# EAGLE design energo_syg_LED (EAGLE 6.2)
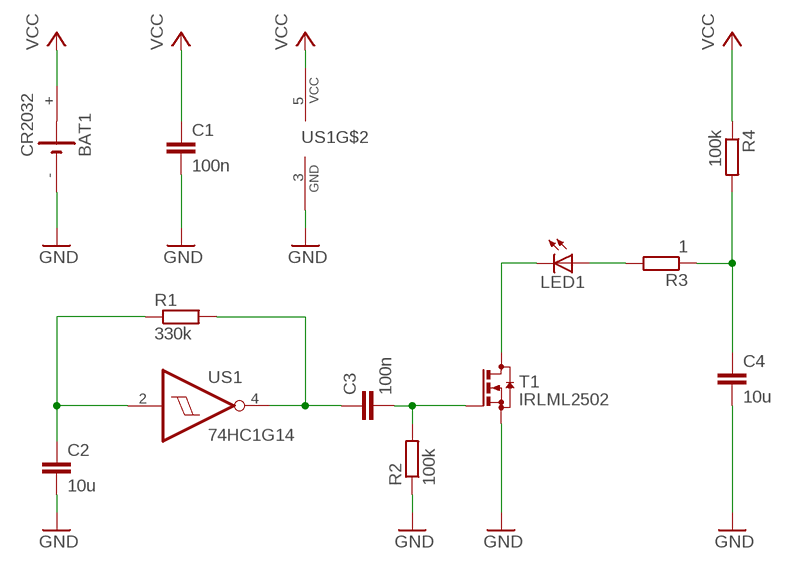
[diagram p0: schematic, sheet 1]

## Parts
BAT1  CR2032  BAT_20/16_XX  [BAT_CR2032]
C1  100n  C-EUC0805  [C0805]
C2  10u  C-EUC0805  [C0805]
C3  100n  C-EUC0805  [C0805]
C4  10u  C-EUC0805  [C0805]
LED1  LED5MM  [LED5MM]
R1  330k  R-EU_R0805  [R0805]
R2  100k  R-EU_R0805  [R0805]
R3  1  R-EU_R0805  [R0805]
R4  100k  R-EU_R0805  [R0805]
T1  IRLML2502  BSS123  [SOT23]
US1  74HC1G14  74LVC1G14  [SOT23-5L]

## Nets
GND: BAT1.- C1.2 C2.2 C4.2 R2.1 T1.2(S) US1.3(GND)
N$1: C3.2 R2.2 T1.1(G)
N$2: C2.1 R1.1 US1.2(I)
N$3: C3.1 R1.2 US1.4(O)
N$4: LED1.K(C) T1.3(D)
N$5: LED1.A R3.2
N$6: C4.1 R3.1 R4.2
VCC: BAT1.+ C1.1 R4.1 US1.5(VCC)

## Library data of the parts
BAT1 = inne_futrzak:BAT_20/16_XX
C1-C4 = rcl:C-EU: CAPACITOR, European symbol
LED1 = led:LED: LED
R1-R4 = rcl:R-EU_: RESISTOR, European symbol
T1 = transistor-small-signal:BSS123: N-CHANNEL MOS FET
US1 = scalaki_futrzak:74LVC1G14

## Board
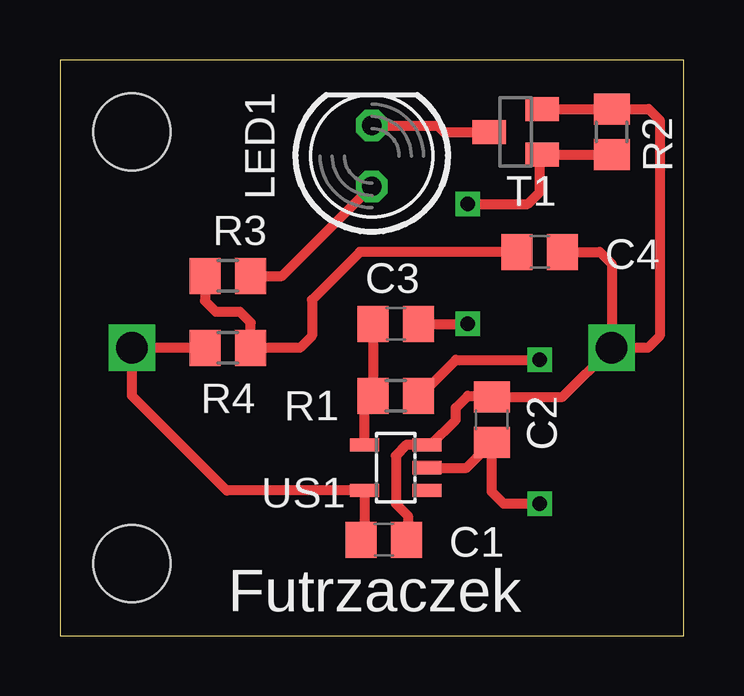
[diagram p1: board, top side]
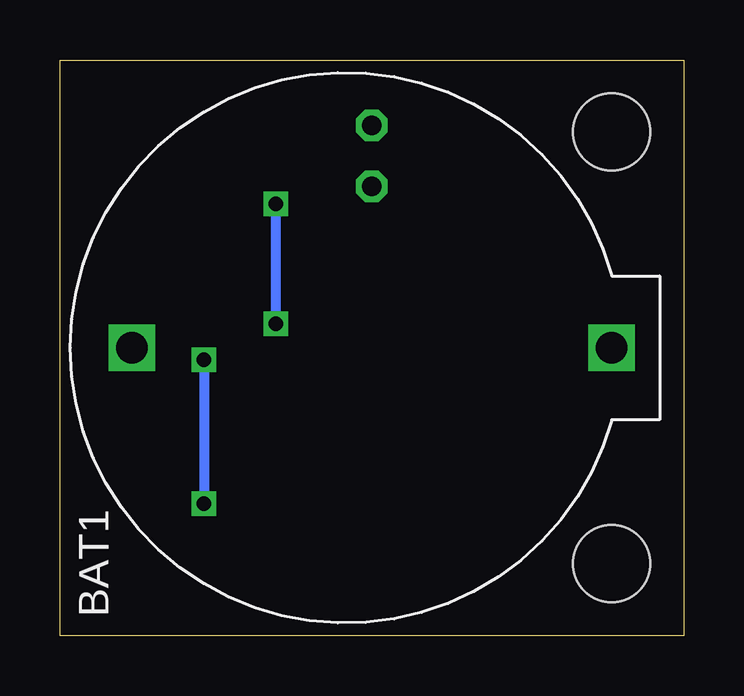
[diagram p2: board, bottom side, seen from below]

Size 26 x 24 mm. Coordinates in mm from the lower left corner, seen from the top.
Outline: 0,0 26,0 26,24 0,24 0,0
Copper layers (1*16): Top 0.035mm / dielectric 1.5mm / Bottom 0.035mm
Design rules: minimum track width 10mil, minimum drill 24mil, track to track 8mil, track to pad 8mil, pad to pad 8mil, via to via 8mil, smd to smd 8mil, copper to edge 40mil, drill to drill 8mil, minimum pad ring 10mil, minimum via ring 8mil, stop-mask expansion 4mil, vias tented up to drill 0mil, thermal gap 10mil
Holes 3.2 mm at 3,3 3,21

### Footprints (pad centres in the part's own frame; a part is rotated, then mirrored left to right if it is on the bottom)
BAT_CR2032 = drill 1.3 square: + 12,0; - -8,0
C0805 = smd 1.3 x 1.5: 1 -0.95,0; 2 0.95,0
LED5MM = drill 0.813 octagon: A -1.27,0; K 1.27,0
R0805 = smd 1.3 x 1.5: 1 -0.95,0; 2 0.95,0
SOT23 = smd 1 x 1.4: 1 -0.95,-1.1; 2 0.95,-1.1; 3 0,1.1
SOT23-5L = smd 0.55 x 1.2: 1 -0.95,-1.3; 2 0,-1.3; 3 0.95,-1.3; 4 0.95,1.3; 5 -0.95,1.3

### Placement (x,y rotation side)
BAT1  15,12 0 bottom
C1  13.5,4 0 top
C2  18,9 90 top
C3  14,13 0 top
C4  20,16 0 top
LED1  13,20 90 top
R1  14,10 180 top
R2  23,21 270 top
R3  7,15 0 top
R4  7,12 0 top
T1  19,21 90 top
US1  14,7 90 top

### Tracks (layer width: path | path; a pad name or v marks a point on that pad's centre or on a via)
GND
  Top 0.406: C1.2 14.5,4.45 14.5,5 14,5.5 14,7.5 14.45,7.95 US1.3 15.45,7.95 16.5,9 16.5,9.5 17,10 17.95,10 C2.2 20.95,9.95 BAT1.- | C4.2 22.5,16 23,15.5 BAT1.- | T1.2 R2.1 24.55,21.95 25,21.5 25,12.5 24.5,12 BAT1.-
N$1  (via drill 0.6)
  Top 0.406: R2.2 T1.1 20,19.95 20,18.5 19.5,18 v17,18 | C3.2 v17,13
  Bottom 0.406: v17,13 v17,18
N$2  (via drill 0.6)
  Top 0.406: US1.2 16.95,7 C2.1 18,6 18.5,5.5 v20,5.5 | R1.1 15,10 16.5,11.5 v20,11.5
  Bottom 0.406: v20,11.5 v20,5.5
N$3
  Top 0.406: US1.4 12.7,9.65 R1.2 C3.1
N$4
  Top 0.406: LED1.K 15.73,21.27 16,21 T1.3
N$5
  Top 0.406: R3.2 9.27,15 LED1.A
N$6
  Top 0.406: R3.1 6.05,13.95 6.5,13.5 7.5,13.5 7.95,13.05 R4.2 10,12 10.5,12.5 10.5,14 12.5,16 C4.1
VCC
  Top 0.406: R4.1 BAT1.+ 3,10 6.95,6.05 US1.5 12.7,4.35 C1.1

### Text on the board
tPlace: Futrzaczek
